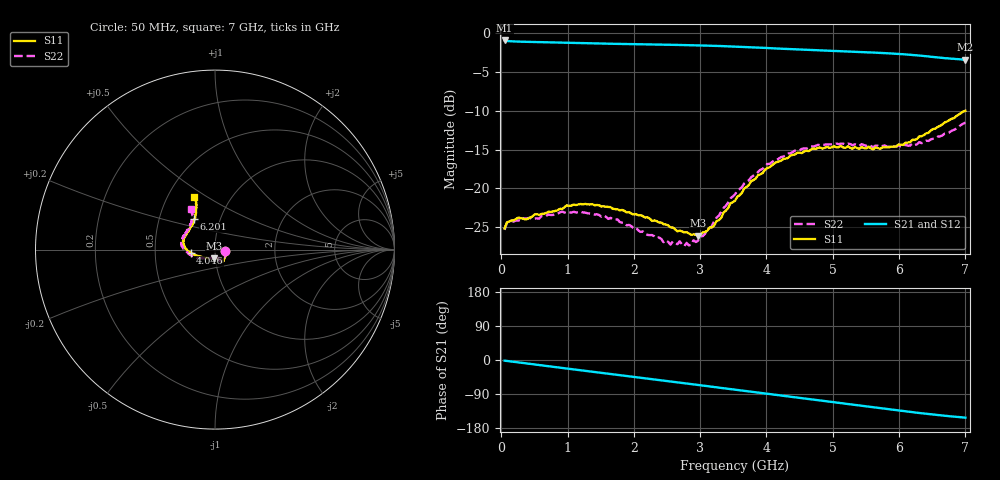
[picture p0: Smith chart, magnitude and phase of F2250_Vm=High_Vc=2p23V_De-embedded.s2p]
! Integrated Device Technology
! Corporate Headquarters
! 6024 Silver Creek Valley Road
! San Jose, CA 95138  USA
! Phone:  1-408-284-8200
! Toll Free:  1-800-223-1366
! Webpage:  http://www.idt.com/
! Timing and RF Division
! 515 Groton Road, Suite 102
! Westford, MA 01886-6024
! Device:  F2250
! Description: Voltage Variable RF Attenuator
! Frequency:  50.0 -  6000.00 MHz
! Package:  3x3 mm Thin QFN Plastic Package: 16 pin
! Ports:  2 RF, 3 DC
!  Pin  1  = GND
!  Pin  2  = NC
!  Pin  3  = RF1  = Port 1
!  Pin  4  = NC
!  Pin  5  = GND
!  Pin  6  = GND
!  Pin  7  = GND
!  Pin  8  = GND
!  Pin  9  = NC
!  Pin 10  = RF2  = Port 2
!  Pin 11  = NC
!  Pin 12  = GND
!  Pin 13  = GND
!  Pin 14  = VCNTRL
!  Pin 15  = VDD
!  Pin 16  = VMODE
! Vcntrl:  2.230 Volts
! Vmode:  +3.300 Volts
! Vdd:  +3.30  Volts
! Current:  1.316 mA
! Data:  The device was measured on a the F2250 evaluation board which has
!  individual transmission lines to the RF pins.  Data was collected
!  using a calibrated network analyzer.  The evaluation board was
!  de-embedded using a TRL calibration technique.
!  The reference plane is the edge of the package pin.
! Misc:  SN 10
!  Action Tracker AT0258
! Date Measured:  2014-11-26
! Date:  2015-10-15  MJV
! Note:
!  Integrated Device Technology supplies this data as a sample of measured
!  data at the package pin for this product.  Your particular data for this
!  product may vary.
!  Data was taken at 25 degrees C.
!  Integrated Device Technology reserves the right to change this data at anytime.
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# GHz S dB R 50
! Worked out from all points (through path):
!   201 points, 50 MHz to 7 GHz, reference 50 ohm
!   highest |S21| = -0.92 dB at 50 MHz (marker M1); lowest = -3.4 dB at 7 GHz (marker M2)
!   group delay of S21, straight-line fit = 61.1 ps
!   lowest |S11| = -26.1 dB at 2.969 GHz (marker M3), VSWR 1.10, Z = 49.3 - j4.89 ohm
!   |S11| at or under -10 dB: start of sweep to 6.994 GHz
!   |S22| runs from -27.4 to -11.5 dB; largest |S21 - S12| = 0.0019
!   S11 on the Smith chart (normalised r, x): 50 MHz: 1.11, -0.02; 4.046 GHz: 0.76, -0.03; 6.201 GHz: 0.75, +0.27; 7 GHz: 0.68, +0.44
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0.05  -25.15 -10.1  -0.92 -1.8  -0.92 -1.8  -25.33 -10.4
0.1195  -24.25 -9.8  -1.02 -3.2  -1.02 -3.2  -24.21 -8.6
0.91875  -22.65 -48.5  -1.21 -21.0  -1.20 -21.1  -22.97 -50.0
1.2315  -22.04 -56.3  -1.27 -27.9  -1.27 -27.9  -23.09 -60.5
1.75275  -22.68 -63.2  -1.36 -39.1  -1.36 -39.1  -23.97 -67.3
2.37825  -24.39 -63.1  -1.45 -52.8  -1.46 -52.8  -26.31 -67.6
2.552  -25.02 -67.8  -1.48 -56.6  -1.48 -56.7  -27.23 -74.1
2.691  -25.44 -75.5  -1.50 -59.7  -1.50 -59.8  -26.80 -81.6
2.7605  -25.67 -77.5  -1.52 -61.3  -1.52 -61.3  -27.43 -85.9
2.969  -26.09 -94.8  -1.56 -66.0  -1.56 -66.0  -26.72 -104.8
3.21225  -24.75 -124.7  -1.61 -71.5  -1.61 -71.5  -24.13 -129.5
3.4555  -21.91 -146.1  -1.69 -76.9  -1.69 -77.0  -21.28 -144.8
3.525  -21.58 -150.5  -1.71 -78.5  -1.71 -78.6  -20.76 -148.0
3.76825  -19.04 -163.1  -1.80 -84.0  -1.80 -84.0  -18.54 -159.1
4.04625  -17.26 -172.7  -1.91 -90.2  -1.91 -90.2  -16.83 -169.5
4.4285  -15.62 177.0  -2.06 -98.6  -2.07 -98.6  -15.11 179.0
4.7065  -14.84 170.0  -2.16 -104.8  -2.16 -104.8  -14.61 173.2
5.054  -14.69 161.8  -2.29 -112.5  -2.29 -112.5  -14.21 166.2
5.85325  -14.68 135.9  -2.59 -130.0  -2.59 -130.1  -14.62 147.4
6.20075  -13.73 124.2  -2.80 -137.7  -2.80 -137.8  -14.21 138.4
6.54825  -12.28 116.1  -3.07 -144.7  -3.07 -144.8  -13.54 127.0
7  -9.98 111.2  -3.40 -152.1  -3.41 -152.2  -11.52 120.7
